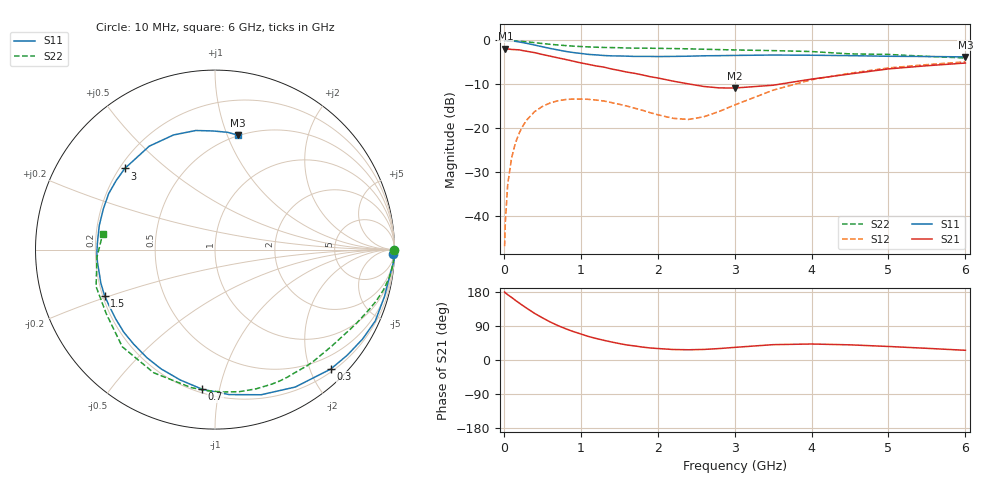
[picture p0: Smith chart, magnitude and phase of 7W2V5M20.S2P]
! Infineon Technologies  Discrete & RF Semiconductors
! BFS17W
! Si NPN RF Bipolar Junction Transistor in SOT323
! VCE = 2.5 V  IC = 0.2 mA
! Common Emitter S-Parameters:  August  1999
# GHz  S  MA  R  50
!  f  S11  S21  S12  S22
! GHz  MAG  ANG  MAG  ANG  MAG  ANG  MAG  ANG
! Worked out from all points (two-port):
!   36 points, 10 MHz to 6 GHz, reference 50 ohm
!   highest |S21| = -1.89 dB at 20 MHz (marker M1); lowest = -10.8 dB at 3 GHz (marker M2)
!   |S21| within 3 dB of the highest: start of sweep to 948.7 MHz
!   lowest |S11| = -3.7 dB at 6 GHz (marker M3), VSWR 4.72, Z = 24.7 + j54.7 ohm
!   |S11| at or under -10 dB: nowhere
!   |S22| runs from -4.0 to 0.0 dB; largest |S21 - S12| = 0.8
!   S11 on the Smith chart (normalised r, x): 10 MHz: 27, -66; 300 MHz: 0.25, -2.34; 700 MHz: 0.22, -0.89; 1.5 GHz: 0.21, -0.19; 3 GHz: 0.22, +0.37; 6 GHz: 0.49, +1.09
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0.01  0.9894 -1.5  0.796 179.3  0.0046 88.3  0.9999 0.0
0.02  0.9999 -3.4  0.804 177.0  0.0087 86.4  0.9946 -1.0
0.05  0.9857 -7.9  0.8 172.4  0.0231 85.3  0.9981 -2.4
0.1  0.9798 -15.4  0.791 165.3  0.0459 80.3  0.9942 -4.7
0.15  0.9776 -24.0  0.786 157.5  0.0682 74.6  0.9897 -7.1
0.2  0.9615 -31.2  0.782 150.3  0.0887 70.5  0.9825 -9.3
0.3  0.9267 -45.9  0.753 136.3  0.1255 61.0  0.9649 -13.5
0.4  0.8868 -59.7  0.727 123.0  0.1554 52.6  0.9439 -17.5
0.5  0.8485 -72.4  0.693 111.5  0.1777 45.3  0.9229 -21.0
0.7  0.7813 -95.2  0.635 91.1  0.2062 33.4  0.8894 -27.4
0.9  0.7293 -114.3  0.582 75.3  0.2157 24.0  0.8621 -33.3
1.1  0.6947 -130.8  0.535 62.1  0.2143 17.0  0.845 -39.1
1.5  0.6666 -157.4  0.456 43.4  0.1884 9.3  0.8269 -51.0
2.2  0.6586 168.3  0.345 27.7  0.1304 22.0  0.809 -73.5
2.6  0.6694 152.2  0.3 27.9  0.1358 45.3  0.7945 -86.9
3  0.6759 138.0  0.288 33.3  0.1848 59.5  0.78 -99.9
3.5  0.6828 122.5  0.31 40.5  0.2724 61.6  0.7665 -116.5
4  0.6793 109.9  0.364 42.2  0.3578 56.1  0.7481 -133.7
4.5  0.6721 99.1  0.416 40.0  0.4239 48.8  0.7035 -149.4
5  0.661 90.9  0.475 35.7  0.4873 41.8  0.6938 -162.7
5.5  0.6573 83.9  0.516 30.8  0.5314 34.9  0.6591 -176.3
6  0.6504 78.6  0.554 25.6  0.5713 28.6  0.6317 171.9
